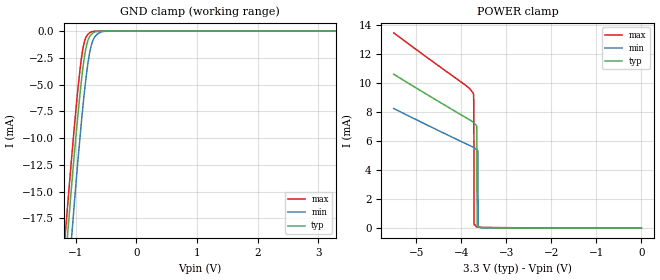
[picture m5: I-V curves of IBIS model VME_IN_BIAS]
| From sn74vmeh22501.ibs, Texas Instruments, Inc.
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[Model]   VME_IN_BIAS
Model_type  Input
Vinl=0.8V
Vinh=2.0V
| variable   typ   min   max
C_comp   2.94pF   2.36pF   3.70pF
[Temperature Range]   40   100   0
| Ambient temperature   25   85   0
[Voltage range]   3.3   3.15   3.45
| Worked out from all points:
|   GND clamp passes 1 mA (typ) near -0.81 V on its own axis
|   POWER clamp passes 1 mA (typ) near -3.65 V on its own axis
[GND Clamp]
| VME_IN_BIAS
|   Voltage   I(typ)   I(min)   I(max)
-5.5V     -380.9mA   -382.8mA   -382.4mA
-1.175V   -21.7mA    -26.84mA   -18.92mA
-1.145V   -19.55mA   -24.62mA   -16.84mA
-1.12V    -17.8mA    -22.78mA   -15.13mA
-1.065V   -14.05mA   -18.82mA   -11.45mA
-945mV    -6.558mA   -10.69mA   -4.224mA
-870mV    -2.818mA   -6.237mA   -1.229mA
-815mV    -1.116mA   -3.549mA   -396.3uA
-760mV    -407.5uA   -1.66mA    -116.4uA
-710mV    -156.5uA   -754.7uA   -24.72uA
-640mV    -24.5uA    -253.6uA   -2.039uA
3.3V      249.2pA    1.317nA    148.6pA
[POWER Clamp]
| VME_IN_BIAS
|   Voltage   I(typ)   I(min)   I(max)
-5.5V     10.59mA    8.234mA    13.43mA
-3.73V    7.267mA    5.557mA    9.25mA
-3.72V    7.238mA    5.538mA    7.795mA
-3.715V   7.223mA    5.528mA    230.4uA
-3.67V    7.078mA    5.431mA    96.79uA
-3.655V   6.993mA    5.395mA    89.22uA
-3.65V    1.83mA     5.383mA    86.88uA
-3.645V   170.1uA    5.371mA    84.61uA
-3.63V    166.3uA    5.291mA    78.26uA
-3.625V   163.8uA    122.5uA    76.3uA
-3.61V    63.88uA    121.7uA    70.87uA
-95.1fV   249.2pA    1.313nA    152.7pA
